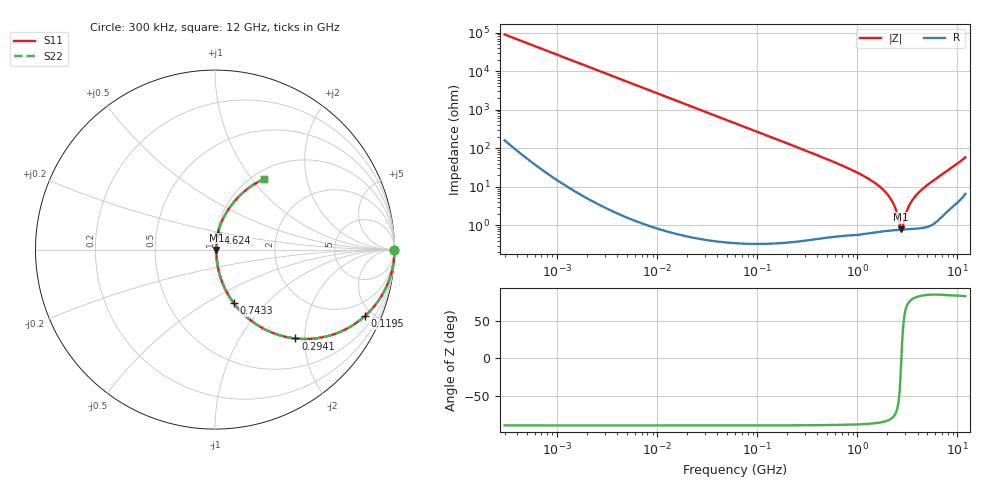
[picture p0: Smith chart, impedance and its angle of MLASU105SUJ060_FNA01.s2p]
! MLASU105SUJ060_FNA01  S-PARAMETER MODEL  ( General Type )
! Model Generated by TAIYO YUDEN Corporation (http://www.ty-top.com)
! Version 2.0
! TAIYO YUDEN Control No. 120810
! Copyright(c) 2012 TAIYO YUDEN CO.,LTD. All Rights Reserved.
! Product Description (link to TY-COMPAS)
! https://ds.yuden.co.jp/TYCOMPAS/or/detail?pn=MLASU105SUJ060DFNA01&u=M
! Products Name : Multilayer Ceramic Capacitors
! Characteristics :
!  Capacitance : 6 pF , Rated Voltage : 50V , TCC : UJ / U2J
!  Case Size : 1.0 x 0.5 / 0.039 x 0.02 [mm/inch] , Thickness : 0.5 / 0.02 [mm/inch]
!  (Conditions: Temperature = 25 degC , DC Bias Current/Voltage = 0A / 0V)
! External Node Assignments :
!  1  o---| |---o  2
! GND o---------o GND
! Frequency Range : 0.3MHz  -  12000MHz  [ 401 STEP ]
# MHz S RI R 50
! Freq[MHz].  S11 Real  S11 Imag  S21 Real  S21 Imag  S12 Real  S12 Imag  S22 Real  S22 Imag
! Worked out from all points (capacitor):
!   401 points, 300 kHz to 12 GHz, reference 50 ohm
!   read as one part in series: C = 5.94 pF near 316.3 kHz
!   lowest |Z| = 796 mohm at 2.722 GHz (marker M1)
!   series resonance near 2.752 GHz, so ESL is about 560 pH
!   S11 on the Smith chart (normalised r, x): 300 kHz: open; 119.5 MHz: 1.01, -4.48; 294.1 MHz: 1.01, -1.80; 743.3 MHz: 1.01, -0.67; 4.624 GHz: 1.02, +0.19; 12 GHz: 1.13, +1.15
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0.3  1 -0.00112  3.26e-06 0.00112  3.26e-06 0.00112  1 -0.00112
1.769972  1 -0.0066  4.62e-05 0.0066  4.62e-05 0.0066  1 -0.0066
10.44266  0.9985 -0.0389  0.00153 0.0389  0.00153 0.0389  0.9985 -0.0389
27.82928  0.9893 -0.1027  0.0107 0.1027  0.0107 0.1027  0.9893 -0.1027
60  0.9521 -0.2131  0.0479 0.2131  0.0479 0.2131  0.9521 -0.2131
119.4772  0.8334 -0.3719  0.1666 0.3719  0.1666 0.3719  0.8334 -0.3719
197.6437  0.6452 -0.4771  0.3548 0.4771  0.3548 0.4771  0.6452 -0.4771
294.0765  0.4484 -0.4951  0.5516 0.4951  0.5516 0.4951  0.4484 -0.4951
353.9943  0.3576 -0.4764  0.6424 0.4764  0.6424 0.4764  0.3576 -0.4764
743.2595  0.1044 -0.2979  0.8956 0.2979  0.8956 0.2979  0.1044 -0.2979
1441.349  0.024 -0.1308  0.976 0.1308  0.976 0.1308  0.024 -0.1308
1781.601  0.0143 -0.0855  0.9857 0.0855  0.9857 0.0855  0.0143 -0.0855
2088.533  0.0101 -0.0534  0.9899 0.0534  0.9899 0.0534  0.0101 -0.0534
2321.999  0.00849 -0.0326  0.9915 0.0326  0.9915 0.0326  0.00849 -0.0326
2650.866  0.00765 -0.00705  0.9923 0.00705  0.9923 0.00705  0.00765 -0.00705
2722.03  0.00764 -0.00199  0.9924 0.00199  0.9924 0.00199  0.00764 -0.00199
2870.14  0.00776 0.00722  0.9922 -0.00722  0.9922 -0.00722  0.00776 0.00722
3190.978  0.00849 0.0256  0.9915 -0.0256  0.9915 -0.0256  0.00849 0.0256
3454.93  0.00949 0.0393  0.9905 -0.0393  0.9905 -0.0393  0.00949 0.0393
4623.766  0.0171 0.0915  0.9829 -0.0915  0.9829 -0.0915  0.0171 0.0915
7854.144  0.0804 0.2321  0.9196 -0.2321  0.9196 -0.2321  0.0804 0.2321
12000  0.2739 0.3927  0.7261 -0.3927  0.7261 -0.3927  0.2739 0.3927
